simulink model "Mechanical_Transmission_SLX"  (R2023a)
settings: Solver=ode23s  StartTime=0.0  StopTime=10.0  MaxStep=0.001  RelTol=1e-3
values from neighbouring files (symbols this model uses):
  b_3 = 2*N/(m/sec)    (= 2)    [Mechanical_Transmission_EQN.m]    (also in Mechanical_Transmission_SLX_m.m; Car_Dumper_EQN.m; Car_Dumper_SLX_m.m; Mechanical_Mass_Spring_Mass_EQN.m)
  b_6 = 2*N/(m/sec)    (= 2)    [Mechanical_Transmission_EQN.m]    (also in Mechanical_Transmission_SLX_m.m; Car_Dumper_EQN.m; Car_Dumper_SLX_m.m; Mechanical_Mass_Spring_Mass_EQN.m)
  b_c = 0.1*Nm/(rad/sec)    (= 0.1)    [Mechanical_Transmission_EQN.m]    (also in Mechanical_Transmission_SLX_m.m)
  b_f = 0.1*Nm/(rad/sec)    (= 0.1)    [Mechanical_Transmission_EQN.m]    (also in Mechanical_Transmission_SLX_m.m)
  F_1_0 = 10*N    (= 10)    [Mechanical_Transmission_SLX_m.m]    (also in Car_Dumper_SLX_m.m; Mechanical_Mass_Spring_Mass_SLX_m.m)
  F_4_0 = 0*N    (= 0)    [Mechanical_Transmission_SLX_m.m]    (also in Car_Dumper_SLX_m.m; Mechanical_Mass_Spring_Mass_SLX_m.m)
  F_7_0 = 0*N    (= 0)    [Mechanical_Transmission_SLX_m.m]
  J_b = 0.01*kg*m^2    (= 0.01)    [Mechanical_Transmission_EQN.m]    (also in Mechanical_Transmission_SLX_m.m)
  J_e = 0.01*kg*m^2    (= 0.01)    [Mechanical_Transmission_EQN.m]    (also in Mechanical_Transmission_SLX_m.m)
  K_4 = 1000*N/m    (= 1000)    [Mechanical_Transmission_EQN.m]    (also in Mechanical_Transmission_SLX_m.m; Car_Dumper_EQN.m; Car_Dumper_SLX_m.m; Mechanical_Mass_Spring_Mass_EQN.m)
  K_7 = 1000*N/m    (= 1000)    [Mechanical_Transmission_EQN.m]    (also in Mechanical_Transmission_SLX_m.m)
  K_d = 10*Nm/rad    (= 10)    [Mechanical_Transmission_EQN.m]    (also in Mechanical_Transmission_SLX_m.m)
  M_2 = 0.5*kg    (= 0.5)    [Mechanical_Transmission_EQN.m]    (also in Mechanical_Transmission_SLX_m.m; Car_Dumper_EQN.m; Car_Dumper_SLX_m.m; Mechanical_Mass_Spring_Mass_EQN.m)
  M_5 = 0.5*kg    (= 0.5)    [Mechanical_Transmission_EQN.m]    (also in Mechanical_Transmission_SLX_m.m; Car_Dumper_EQN.m; Car_Dumper_SLX_m.m; Mechanical_Mass_Spring_Mass_EQN.m)
  R = 1    [Mechanical_Transmission_EQN.m]    (also in Mechanical_Transmission_SLX_m.m; Electrical_Transformer_EQN.m; Electrical_Transformer_SLX_m.m; Mechanical_system_EQN.m)
  T_d_0 = 0*Nm    (= 0)    [Mechanical_Transmission_SLX_m.m]
  T_g_0 = 0*Nm    (= 0)    [Mechanical_Transmission_SLX_m.m]
  Ts = Tfin/Nr_Ts_Points    (= 0.0014747)    [Mechanical_Transmission_SLX_m.m]    (also in BIG_EC_Simscape_SLX_m.m = 0.0003; Car_Dumper_SLX_m.m = 0.0022779; Electric_Circuit_01_SLX_m.m = 0.005; Electric_Circuit_02_SLX_m.m = 0.000480145)
  v_2_0 = 0*m/sec    (= 0)    [Mechanical_Transmission_SLX_m.m]    (also in Car_Dumper_SLX_m.m; Mechanical_Mass_Spring_Mass_SLX_m.m)
  v_5_0 = 0*m/sec    (= 0)    [Mechanical_Transmission_SLX_m.m]    (also in Car_Dumper_SLX_m.m; Mechanical_Mass_Spring_Mass_SLX_m.m)
  w_b_0 = 0*rad/sec    (= 0)    [Mechanical_Transmission_SLX_m.m]
  w_e_0 = 0*rad/sec    (= 0)    [Mechanical_Transmission_SLX_m.m]

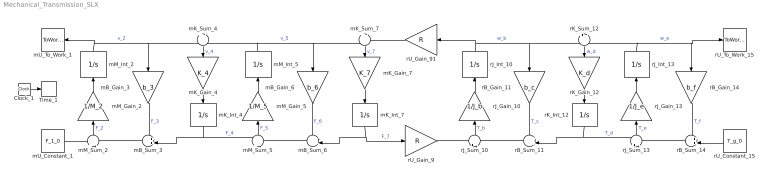
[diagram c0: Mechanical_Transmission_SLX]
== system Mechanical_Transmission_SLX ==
  Clock_1 : Clock
  Time_1 : ToWorkspace  VariableName=t  SaveFormat=Timeseries  SampleTime=Ts
  mB_Gain_3 : Gain  Gain=b_3  Multiplication=Matrix(K*u)
  mB_Gain_6 : Gain  Gain=b_6  Multiplication=Matrix(K*u)
  mB_Sum_3 : Sum  Inputs=++|
  mB_Sum_6 : Sum  Inputs=++|
  mK_Gain_4 : Gain  Gain=K_4  Multiplication=Matrix(K*u)
  mK_Gain_7 : Gain  Gain=K_7  Multiplication=Matrix(K*u)
  mK_Int_4 : Integrator  InitialCondition=F_4_0
  mK_Int_7 : Integrator  InitialCondition=F_7_0
  mK_Sum_4 : Sum  Inputs=+|-
  mK_Sum_7 : Sum  Inputs=+|-
  mM_Gain_2 : Gain  Gain=1/M_2  Multiplication=Matrix(K*u)
  mM_Gain_5 : Gain  Gain=1/M_5  Multiplication=Matrix(K*u)
  mM_Int_2 : Integrator  InitialCondition=v_2_0
  mM_Int_5 : Integrator  InitialCondition=v_5_0
  mM_Sum_2 : Sum  Inputs=+|-
  mM_Sum_5 : Sum  Inputs=+|-
  mU_Constant_1 : Constant  Value=F_1_0
  mU_To_Work_1 : ToWorkspace  VariableName=v_1_0  SaveFormat=Timeseries  SampleTime=Ts
  rB_Gain_11 : Gain  Gain=b_c  Multiplication=Matrix(K*u)
  rB_Gain_14 : Gain  Gain=b_f  Multiplication=Matrix(K*u)
  rB_Sum_11 : Sum  Inputs=++|
  rB_Sum_14 : Sum  Inputs=++|
  rJ_Gain_10 : Gain  Gain=1/J_b  Multiplication=Matrix(K*u)
  rJ_Gain_13 : Gain  Gain=1/J_e  Multiplication=Matrix(K*u)
  rJ_Int_10 : Integrator  InitialCondition=w_b_0
  rJ_Int_13 : Integrator  InitialCondition=w_e_0
  rJ_Sum_10 : Sum  Inputs=+|-
  rJ_Sum_13 : Sum  Inputs=+|-
  rK_Gain_12 : Gain  Gain=K_d  Multiplication=Matrix(K*u)
  rK_Int_12 : Integrator  InitialCondition=T_d_0
  rK_Sum_12 : Sum  Inputs=+|-
  rU_Constant_15 : Constant  Value=T_g_0
  rU_Gain_9 : Gain  Gain=R  Multiplication=Matrix(K*u)
  rU_Gain_91 : Gain  Gain=R  Multiplication=Matrix(K*u)
  rU_To_Work_15 : ToWorkspace  VariableName=w_g_0  SaveFormat=Timeseries  SampleTime=Ts
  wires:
  mU_Constant_1/1 -> mM_Sum_2/1
  mB_Sum_3/1 -> mM_Sum_2/2
  mM_Int_2/1 -> mU_To_Work_1/1, mB_Gain_3/1, mK_Sum_4/1  "v_2"
  mM_Sum_2/1 -> mM_Gain_2/1  "F_2"
  mM_Gain_2/1 -> mM_Int_2/1
  mK_Int_4/1 -> mB_Sum_3/2, mM_Sum_5/1  "F_4"
  mB_Gain_3/1 -> mB_Sum_3/1  "F_3"
  mM_Int_5/1 -> mK_Sum_4/2, mB_Gain_6/1, mK_Sum_7/1  "v_5"
  mK_Sum_4/1 -> mK_Gain_4/1  "v_4"
  mK_Gain_4/1 -> mK_Int_4/1
  mB_Sum_6/1 -> mM_Sum_5/2
  mM_Sum_5/1 -> mM_Gain_5/1  "F_5"
  mM_Gain_5/1 -> mM_Int_5/1
  mK_Int_7/1 -> mB_Sum_6/2, rU_Gain_9/1  "F_7"
  mB_Gain_6/1 -> mB_Sum_6/1  "F_6"
  rU_Gain_91/1 -> mK_Sum_7/2
  mK_Sum_7/1 -> mK_Gain_7/1  "v_7"
  mK_Gain_7/1 -> mK_Int_7/1
  rU_Gain_9/1 -> rJ_Sum_10/1
  rJ_Int_10/1 -> rU_Gain_91/1, rB_Gain_11/1, rK_Sum_12/1  "w_b"
  rB_Sum_11/1 -> rJ_Sum_10/2
  rJ_Sum_10/1 -> rJ_Gain_10/1  "T_b"
  rJ_Gain_10/1 -> rJ_Int_10/1
  rK_Int_12/1 -> rB_Sum_11/2, rJ_Sum_13/1  "T_d"
  rB_Gain_11/1 -> rB_Sum_11/1  "T_c"
  rJ_Int_13/1 -> rK_Sum_12/2, rU_To_Work_15/1, rB_Gain_14/1  "w_e"
  rK_Sum_12/1 -> rK_Gain_12/1  "w_d"
  rK_Gain_12/1 -> rK_Int_12/1
  rB_Sum_14/1 -> rJ_Sum_13/2
  rJ_Sum_13/1 -> rJ_Gain_13/1  "T_e"
  rJ_Gain_13/1 -> rJ_Int_13/1
  rU_Constant_15/1 -> rB_Sum_14/2
  rB_Gain_14/1 -> rB_Sum_14/1  "T_f"
  Clock_1/1 -> Time_1/1
